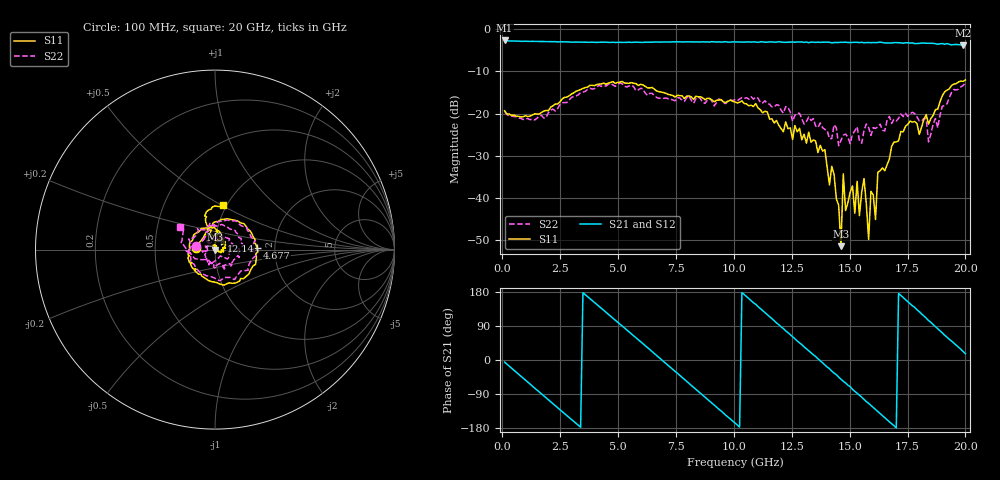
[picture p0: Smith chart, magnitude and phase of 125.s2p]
!Agilent Technologies,N5230C,MY49001569,A.09.33.09
!Agilent N5230C: A.09.33.09
!Date: Sunday, July 26, 2015 15:18:29
!Correction: S11(Full 2 Port(1,2))
!S21(Full 2 Port(1,2))
!S12(Full 2 Port(1,2))
!S22(Full 2 Port(1,2))
!S2P File: Measurements: S11, S21, S12, S22:
# Hz S  dB  R 50
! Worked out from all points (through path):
!   201 points, 100 MHz to 20 GHz, reference 50 ohm
!   highest |S21| = -2.65 dB at 100 MHz (marker M1); lowest = -3.8 dB at 19.9 GHz (marker M2)
!   group delay of S21, straight-line fit = 147 ps
!   lowest |S11| = -51.4 dB at 14.63 GHz (marker M3), VSWR 1.01, Z = 50.3 + j0.00139 ohm
!   |S11| at or under -10 dB: start of sweep to end of sweep
!   |S22| runs from -27.6 to -12.7 dB; largest |S21 - S12| = 0.031
!   S11 on the Smith chart (normalised r, x): 100 MHz: 0.81, +0.01; 4.677 GHz: 1.61, +0.02; 12.14 GHz: 1.07, +0.11; 20 GHz: 0.97, +0.51
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1e8  -19.35 175.2  -2.65 -5.6  -2.66 -5.9  -19.58 169.5
1.7915e9  -19.41 116.9  -2.92 -94.6  -2.93 -94.7  -21.04 127.8
3.483e9  -14.04 55.2  -3.07 177.6  -3.09 177.4  -14.91 65.9
4.677e9  -12.61 1.7  -3.12 115.6  -3.10 115.6  -12.77 12.8
6.7665e9  -14.80 -89.6  -3.06 6.6  -3.03 6.6  -16.39 -101.6
8.3585e9  -15.88 -153.4  -3.01 -77.3  -2.96 -77.7  -16.50 161.2
1.005e10  -17.25 134.6  -2.99 -166.3  -3.06 -166.8  -16.73 66.1
1.21395e10  -24.33 55.5  -3.08 83.0  -3.05 82.6  -19.91 -61.7
1.3433e10  -26.25 -16.1  -3.06 14.0  -3.18 13.4  -21.19 -116.2
1.43285e10  -34.46 -28.8  -3.14 -34.4  -3.03 -34.6  -22.67 -174.1
1.4627e10  -51.45 0.3  -3.07 -50.7  -3.07 -50.3  -26.33 158.5
1.47265e10  -34.30 -29.4  -3.10 -56.2  -3.09 -55.7  -25.13 155.4
1.5423e10  -44.20 59.1  -3.17 -92.8  -3.22 -92.9  -26.45 134.4
1.5622e10  -35.42 5.7  -3.20 -103.8  -3.15 -103.4  -24.03 98.9
1.5821e10  -49.85 125.3  -3.14 -114.2  -3.21 -114.7  -23.27 111.5
1.59205e10  -38.45 68.1  -3.19 -119.8  -3.16 -120.8  -25.18 103.5
1.61195e10  -45.12 61.8  -3.18 -130.6  -3.25 -130.7  -23.53 75.5
1.6219e10  -33.93 101.4  -3.13 -136.0  -3.16 -135.9  -23.11 82.5
1.67165e10  -30.78 92.7  -3.26 -162.9  -3.24 -163.6  -20.67 62.4
1.8408e10  -22.51 94.0  -3.33 104.1  -3.23 104.3  -26.70 -49.5
1.99005e10  -12.36 84.6  -3.82 22.3  -3.74 22.2  -13.35 148.8
2e10  -12.02 79.1  -3.69 16.7  -3.83 16.4  -12.72 147.6
